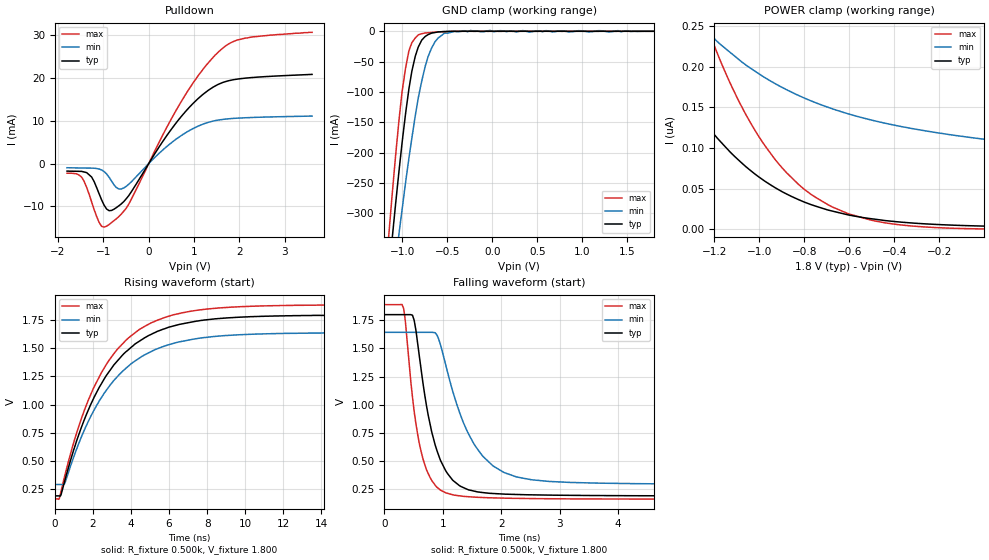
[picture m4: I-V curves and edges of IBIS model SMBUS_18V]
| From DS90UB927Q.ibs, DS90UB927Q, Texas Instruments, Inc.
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|   Model
[Model] SMBUS_18V
Model_type Open_sink
Enable Active-High
Vmeas = 0.9V
Cref = 0.0pF
Rref = 1.0e10
Vref = 0.0V
C_comp   7.2pF   6.2pF   8.2pF
[Voltage Range]   1.8V   1.62V   1.98V
[Temperature Range]   25.0   130.0   -40.0
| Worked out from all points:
|   slope of the pulldown table from 0 to 0.27 V, typ, clamps not added: 59.4 ohm
|   GND clamp passes 1 mA (typ) near -0.59 V on its own axis
|   rising waveform, R_fixture 0.500k, V_fixture 1.800: 20-80 % time 2.95ns typ, 3.04ns min, 2.84ns max; typ from 0.189 V to 1.8 V
|   falling waveform, R_fixture 0.500k, V_fixture 1.800: 20-80 % time 370ps typ, 620ps min, 275ps max; typ from 1.8 V to 0.189 V
[GND Clamp]
-1.8V     -1.522A    -1.361A    -1.657A
-1.148V   -393.4mA   -469mA     -327.6mA
-1.115V   -341.9mA   -427.7mA   -269.2mA
-1.076V   -284.3mA   -379.6mA   -204.6mA
-1.038V   -229.2mA   -332.6mA   -145.3mA
-966.7mV  -136.8mA   -250.6mA   -61.53mA
-895.4mV  -65.54mA   -175.9mA   -18.68mA
-824.2mV  -25.79mA   -109.6mA   -5.932mA
-714.5mV  -5.439mA   -41.38mA   -2.413mA
-637.8mV  -2.003mA   -17.21mA   -1.418mA
-533.6mV  -465.9uA   -3.017mA   -580.1uA
1.796V    -1.298uA   0A         29.56uA
[POWER Clamp]
-1.8V     461.9nA    607.5nA    6.385uA
-1.493V   247nA      340.5nA    497.2nA
-1.367V   182.2nA    287nA      365nA
-1.241V   130.8nA    246.3nA    256.2nA
-1.219V   123.1nA    240.1nA    239.7nA
-1.131V   95.79nA    218.2nA    181.1nA
-1.022V   68.72nA    195.1nA    123.1nA
-928.3mV  51.18nA    179.2nA    85.66nA
-857.1mV  40.68nA    168.9nA    64.02nA
-692.6mV  23.76nA    150nA      30.16nA
-511.7mV  13.54nA    135.2nA    12.15nA
-1.827mV  4.12nA     111nA      623.8pA
[Pulldown]
-1.8V     -1.759mA   -966.5uA   -2.249mA
-1.477V   -1.82mA    -1.026mA   -3.176mA
-1.257V   -3.148mA   -1.062mA   -8.973mA
-1.093V   -7.057mA   -1.265mA   -13.74mA
-928.3mV  -10.6mA    -2.412mA   -14.62mA
-714.5mV  -10.29mA   -5.58mA    -12.9mA
-550.1mV  -8.872mA   -5.69mA    -11.12mA
705.4mV   10.84mA    6.466mA    14.28mA
1.199V    16.19mA    9.225mA    22.06mA
1.577V    18.71mA    10.24mA    26.47mA
2.125V    19.95mA    10.7mA     29.29mA
3.6V      20.83mA    11.1mA     30.65mA
[Rising Waveform]
R_fixture = 0.500k
V_fixture = 1.800
V_fixture_min = 1.620
V_fixture_max = 1.980
|  time   V(typ)   V(min)   V(max)
0s        188.6mV    289.3mV    160.9mV
240ps     187.7mV    289.3mV    165.6mV
510ps     313.2mV    294.7mV    356.9mV
1.5ns     842.9mV    752.7mV    924.4mV
2.43ns    1.179V     1.057V     1.278V
3.81ns    1.479V     1.333V     1.584V
5.64ns    1.666V     1.512V     1.767V
7.83ns    1.751V     1.595V     1.845V
10.8ns    1.784V     1.627V     1.876V
30ns      1.797V     1.643V     1.889V
[Falling Waveform]
R_fixture = 0.500k
V_fixture = 1.800
V_fixture_min = 1.620
V_fixture_max = 1.980
|  time   V(typ)   V(min)   V(max)
0s        1.8V       1.643V     1.889V
330ps     1.8V       1.643V     1.853V
480ps     1.795V     1.643V     1.066V
660ps     1.19V      1.643V     519mV
870ps     641mV      1.639V     285.6mV
1.05ns    414.1mV    1.352V     218.6mV
1.32ns    272.3mV    885.6mV    189.2mV
1.86ns    212.5mV    457.5mV    173.7mV
3.12ns    196.4mV    311.8mV    165.2mV
30ns      188.9mV    289.3mV    160.9mV
[Ramp]
R_load = 500.0
dV/dt_r   9.652376E-1/2.97E-9   8.126717E-1/3.06E-9   1.086925E0/2.85E-9
dV/dt_f   9.666394E-1/3.6E-10   8.145621E-1/6.3E-10   1.088905E0/2.7E-10
